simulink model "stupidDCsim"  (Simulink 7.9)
settings: Solver=ode45  SolverMode=SingleTasking  StartTime=0.0  StopTime=100  RelTol=1e-3  AbsTol=1e-6
PreLoadFcn:
  | stupidDCinit
InitFcn:
  | stupidDCinit
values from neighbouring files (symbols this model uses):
  Ts = 0.1    [stupidDCinit.m]    (also in pidDCinit.m; da_bode_evolution.m = 1)
undefined symbols (not defined in the file or in its folder): conv, polyc2d, polyval
libraries: adaptlib x3, simulink x1

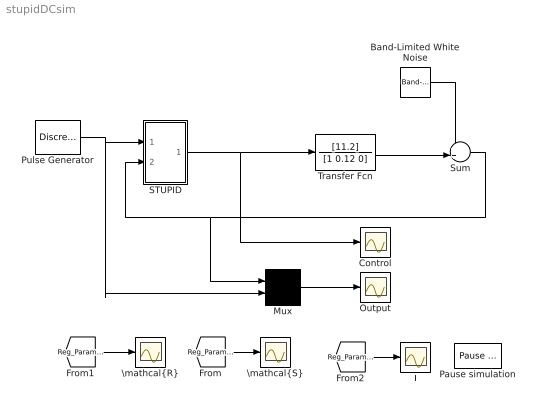
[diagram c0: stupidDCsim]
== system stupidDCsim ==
  Band-Limited White Noise : simulink/Sources/Band-Limited White Noise  Cov=[0.0001]  Ts=0.1  seed=[23341]
  Control : Scope
  Mux : Mux  Inputs=2
  Output : Scope
  Pause simulation : adaptlib/Pause simulation  par=[50]
  Pulse Generator : DiscretePulseGenerator  PulseType=Time based  Amplitude=2  Period=10  PulseWidth=50
  STUPID : Subsystem  mask{wo=5, zeta=1, theta0=[0.3;0.1;2; -2], P0=1000*diag([1 1 1 1]), lambda=.999, a_o=.5, h=Ts, d0=1, um=10}
      mask prompts: wo "w_o (closed loop bandwidth)"; zeta "Closed loop damping"; theta0 "Initial estimate"; P0 "Initial covariance matrix"; lambda "Forgeting factor"; a_o "Observer pole"; h "Sampling time"; d0 "d0 (prediction horizon)"; um "Maximum control signal"
      mask help: DSTR with integral term.
      mask init:
      | Ts=0.1;
  Sum : Sum  Inputs=++|
  T : Scope
  Transfer Fcn : TransferFcn  Numerator=[11.2]  Denominator=[1 0.12 0]
  "\\mathcal{R}" : Scope
  "\\mathcal{S}" : Scope
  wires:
  Mux/1 -> Output/1
  Pulse Generator/1 -> Mux/2, STUPID/1(u_c)
  STUPID/1(u) -> Control/1, Transfer Fcn/1
  Transfer Fcn/1 -> Sum/2
  Sum/1 -> STUPID/2(y), Mux/1
  Band-Limited White Noise/1 -> Sum/1
  [Reg_ParametersStilde] -> "\\mathcal{S}"/1
  [Reg_ParametersRtilde] -> "\\mathcal{R}"/1
  [Reg_ParametersT] -> T/1

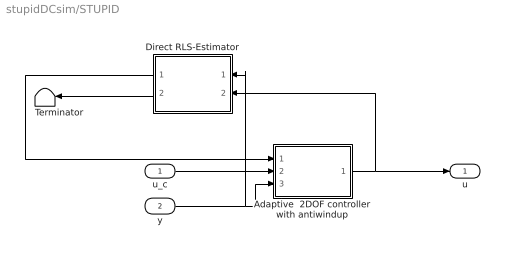
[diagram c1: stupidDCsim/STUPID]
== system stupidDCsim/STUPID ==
  u_c : Inport
  y : Inport  Port=2
  Adaptive  2DOF controller with antiwindup : Subsystem  AncestorBlock=|  mask{n_r=2, ulim=um, A_m=polyc2d([1 2*zeta*wo wo^2],h), A_o=[1 -a_o], A_ow=polyc2d([1 2*0.7*7 7^2],h), h=h}
      | adaptlib/Adaptive 
      | 2DOF controller
      | with antiwindup
      mask prompts: n_r "n_r (degree of R, S and T)"; ulim "Maximum control signal"; A_o "A_o (Observer polynomial)"; A_ow "A_ow (Anti windup polynomial)"; h "Sampling period"
      mask help: A two-degree-of-freedom linear controller with control signal saturation and anti windup. A_o(q)v(k)=T(q)u_c(k)-S(q)y(k)-(A_o(q)-R(q))u(t) u(k)=f(v(k))
  Direct RLS-Estimator : Subsystem  Priority=1  AncestorBlock=adaptlib/Direct RLS-Estimator  mask{n_r=1, theta_0=theta0, P_0=P0, lambda=lambda, A_m=polyc2d([1 2*zeta*wo wo^2],h), A_o=[1 -a_o], d0=d0, h=h}
      mask prompts: n_r "n_r (degree of estimated R, S )"; theta_0 "Initial estimate"; P_0 "Initial covariance matrix"; h "Sampling period"
  Terminator : Terminator
  u : Outport
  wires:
  Direct RLS-Estimator/2(P) -> Terminator/1
  Direct RLS-Estimator/1("[R,S,T]") -> Adaptive  2DOF controller with antiwindup/1("[R,S,T]")
  u_c/1 -> Adaptive  2DOF controller with antiwindup/2(u_c)
  y/1 -> Adaptive  2DOF controller with antiwindup/3(y), Direct RLS-Estimator/1(y)
  Adaptive  2DOF controller with antiwindup/1(u) -> Direct RLS-Estimator/2(u), u/1

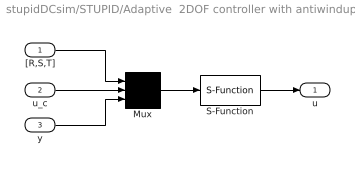
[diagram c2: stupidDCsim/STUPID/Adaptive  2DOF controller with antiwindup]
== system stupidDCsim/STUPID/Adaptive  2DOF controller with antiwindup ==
  "[R,S,T]" : Inport
  u_c : Inport  Port=2
  y : Inport  Port=3
  Mux : Mux  Inputs=3
  S-Function : S-Function  FunctionName=rstdirint  Parameters=2,h,A_o,A_ow,A_m,ulim  EnableBusSupport=off
  u : Outport  InitialOutput=0
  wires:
  "[R,S,T]"/1 -> Mux/1
  y/1 -> Mux/3
  Mux/1 -> S-Function/1
  S-Function/1 -> u/1
  u_c/1 -> Mux/2

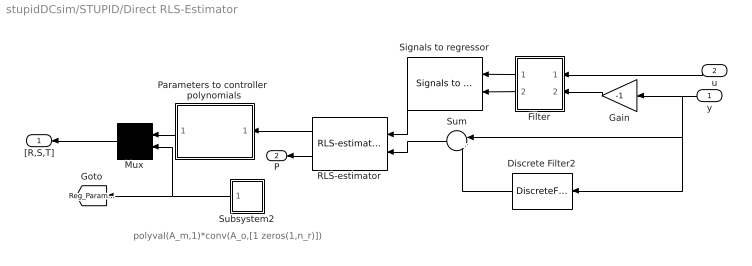
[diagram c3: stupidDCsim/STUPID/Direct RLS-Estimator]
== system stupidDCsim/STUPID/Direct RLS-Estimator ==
  note: polyval(A_m,1)*conv(A_o,[1 zeros(1,n_r)])
  y : Inport
  u : Inport  Port=2
  Discrete Filter2 : DiscreteFilter  Numerator=[zeros(1,d0) 1]*polyval(A_m,1)*polyval(A_o,1)  Denominator=conv(A_m,A_o)  SampleTime=h
  Filter : Subsystem  mask{A_m=A_m, A_o=A_o, d0=d0, h=h}
  Gain : Gain  Gain=-1
  Mux : Mux  Inputs=2
  Parameters to controller  polynomials : Subsystem  AncestorBlock="adaptlib/Parameters to controller  polynomials"  mask{n_r=n_r}
      mask prompts: n_r "n_r (degree of R, S )"
  RLS-estimator : adaptlib/RLS-estimator  n=2*(n_r+1)  theta_0=theta_0  P_0=P_0  lambda=lambda  h=h
  Signals to regressor : adaptlib/Signals to regressor  m=n_r+1  n=n_r+1  h=h
  Subsystem2 : Subsystem
  Sum : Sum  Inputs=|+-
  "[R,S,T]" : Outport  InitialOutput=0
  P : Outport  Port=2  InitialOutput=0
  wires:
  Mux/1 -> "[R,S,T]"/1
  Gain/1 -> Filter/2(y)
  u/1 -> Filter/1(u)
  y/1 -> Gain/1, Sum/1, Discrete Filter2/1
  Filter/1(u_f) -> Signals to regressor/1
  Filter/2(y_f) -> Signals to regressor/2
  Signals to regressor/1 -> RLS-estimator/1
  RLS-estimator/2 -> P/1
  RLS-estimator/1 -> Parameters to controller  polynomials/1(theta)
  Parameters to controller  polynomials/1("[R,S]") -> Mux/1
  Sum/1 -> RLS-estimator/2
  Discrete Filter2/1 -> Sum/2
  Subsystem2/1(Out1) -> Mux/2, [Reg_ParametersT]

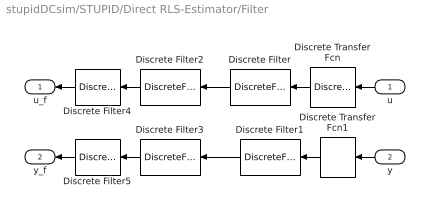
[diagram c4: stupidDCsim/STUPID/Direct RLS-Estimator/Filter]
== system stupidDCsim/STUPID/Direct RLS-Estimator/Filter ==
  u : Inport
  y : Inport  Port=2
  Discrete Transfer Fcn : DiscreteTransferFcn  Denominator=[1 zeros(1,d0) ]  SampleTime=h
  Discrete Transfer Fcn1 : DiscreteTransferFcn  Denominator=[1 zeros(1,d0) ]  SampleTime=h
  Discrete Filter : DiscreteFilter  Denominator=A_o  SampleTime=h
  Discrete Filter1 : DiscreteFilter  Denominator=A_o  SampleTime=h
  Discrete Filter2 : DiscreteFilter  Denominator=A_m  SampleTime=h
  Discrete Filter3 : DiscreteFilter  Denominator=A_m  SampleTime=h
  Discrete Filter4 : DiscreteFilter  Numerator=[1 -1]  Denominator=[1]  SampleTime=h
  Discrete Filter5 : DiscreteFilter  Numerator=[1 -1]  Denominator=[1 ]  SampleTime=h
  u_f : Outport  InitialOutput=0
  y_f : Outport  Port=2  InitialOutput=0
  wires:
  Discrete Filter2/1 -> Discrete Filter4/1
  Discrete Filter3/1 -> Discrete Filter5/1
  u/1 -> Discrete Transfer Fcn/1
  y/1 -> Discrete Transfer Fcn1/1
  Discrete Filter/1 -> Discrete Filter2/1
  Discrete Filter1/1 -> Discrete Filter3/1
  Discrete Transfer Fcn/1 -> Discrete Filter/1
  Discrete Transfer Fcn1/1 -> Discrete Filter1/1
  Discrete Filter4/1 -> u_f/1
  Discrete Filter5/1 -> y_f/1

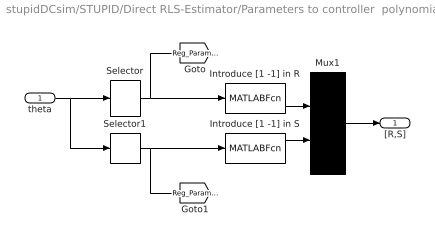
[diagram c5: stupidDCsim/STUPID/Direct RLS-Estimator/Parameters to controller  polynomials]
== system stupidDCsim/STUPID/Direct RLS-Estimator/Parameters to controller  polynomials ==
  theta : Inport
  Introduce [1 -1] in R : MATLABFcn  MATLABFcn=conv(u,[1 -1])  OutputDimensions=3
  Introduce [1 -1] in S : MATLABFcn  MATLABFcn=conv(u,[1 -1])  OutputDimensions=3
  Mux1 : Mux  Inputs=2
  Selector : Selector  InputPortWidth=2*(n_r+1)  IndexOptions=Index vector (dialog)  Indices=[1 : n_r+1]  OutputSizes=1
  Selector1 : Selector  InputPortWidth=2*(n_r+1)  IndexOptions=Index vector (dialog)  Indices="[n_r+2 :  2*(n_r+1)]"  OutputSizes=1
  "[R,S]" : Outport  InitialOutput=0
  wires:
  Selector1/1 -> Introduce [1 -1] in S/1, [Reg_ParametersStilde]
  Mux1/1 -> "[R,S]"/1
  Selector/1 -> Introduce [1 -1] in R/1, [Reg_ParametersRtilde]
  theta/1 -> Selector/1, Selector1/1
  Introduce [1 -1] in R/1 -> Mux1/1
  Introduce [1 -1] in S/1 -> Mux1/2

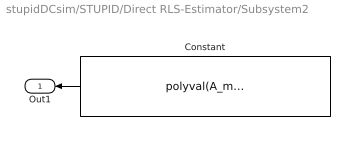
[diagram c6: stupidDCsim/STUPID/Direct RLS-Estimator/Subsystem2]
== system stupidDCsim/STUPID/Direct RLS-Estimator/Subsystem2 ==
  Constant : Constant  Value=polyval(A_m,1)*conv(A_o,[1 zeros(1,n_r)])
  Out1 : Outport
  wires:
  Constant/1 -> Out1/1
